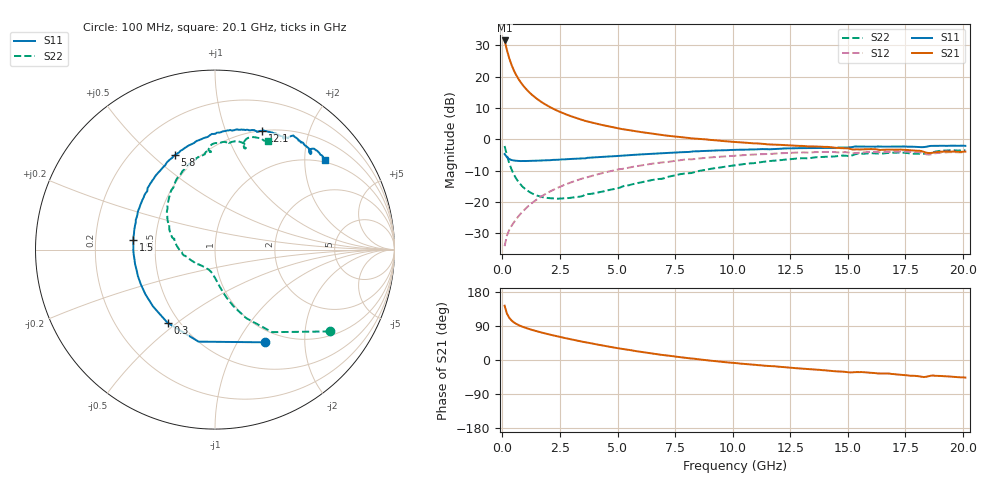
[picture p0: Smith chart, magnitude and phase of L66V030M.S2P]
!  Infineon Technologies AG
! BFR380L3 , PF131585-7, No.6, Th 09.10.01, soldered on pcb-board, measured with PP GSG850
!  Vce=6.0 V,  Ic=30.0 mA
! Common Emitter S-Parameters:  15. November 2001
#  GHz  S  MA  R  50
! f  S11  S21  S12  S22
! GHz  Mag  Ang  Mag  Ang  Mag  Ang  Mag  Ang
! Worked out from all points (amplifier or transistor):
!   201 points, 100 MHz to 20.1 GHz, reference 50 ohm
!   highest |S21| = 31.6 dB at 100 MHz (marker M1)
!   |S21| within 3 dB of that: start of sweep to 198.6 MHz
!   unconditionally stable (mu >= 1): 1.287 GHz to 4.334 GHz
!   at 3.4 GHz: K = 1.02, MAG = 8.7 dB, |S12| = -12.7 dB
!   at 10.1 GHz: K = 0.95, MSG = 2.2 dB, |S12| = -5.2 dB
!   at 20.1 GHz: K = 0.98, MSG = 0.1 dB, |S12| = -4.1 dB
!   S11 on the Smith chart (normalised r, x): 100 MHz: 0.83, -1.31; 300 MHz: 0.43, -0.46; 1.5 GHz: 0.37, +0.05; 5.8 GHz: 0.38, +0.59; 12.1 GHz: 0.50, +1.35; 20.1 GHz: 0.94, +2.51
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0.1  0.5856 -61.9  38.01 143.4  0.01977 63.3  0.7855 -35.5
0.2  0.5209 -100.1  26.78 122.6  0.02924 56.4  0.5593 -55.3
0.3  0.486 -123.0  19.81 111.5  0.03579 56.0  0.4181 -65.6
0.4  0.4685 -137.5  15.52 104.4  0.04163 57.1  0.3319 -71.9
0.5  0.4607 -147.4  12.68 99.3  0.04727 58.9  0.2762 -76.4
0.6  0.4562 -155.1  10.7 95.6  0.05313 60.4  0.2382 -79.6
0.7  0.4542 -161.0  9.258 92.4  0.05923 61.7  0.2101 -82.5
0.8  0.4515 -165.5  8.147 89.6  0.06541 63.0  0.1894 -84.9
1  0.4519 -173.3  6.582 85.0  0.07798 64.4  0.1611 -89.2
1.2  0.455 -179.4  5.519 81.1  0.09076 65.2  0.1435 -93.3
1.5  0.458 173.2  4.455 75.8  0.1103 65.5  0.1273 -99.3
1.8  0.4624 167.0  3.743 71.0  0.1299 65.0  0.1185 -105.5
2.3  0.4718 157.8  2.975 63.7  0.1624 63.3  0.1132 -116.5
2.8  0.4836 149.7  2.484 56.9  0.1946 60.9  0.1154 -126.9
3.5  0.498 139.6  2.029 48.0  0.2394 56.9  0.1254 -139.1
5.8  0.572 113.0  1.352 23.5  0.3723 42.4  0.1983 -179.9
6.8  0.5996 103.5  1.195 14.5  0.4242 35.3  0.2338 166.1
10.1  0.6806 79.0  0.9095 -8.0  0.5508 13.8  0.3869 131.4
12.1  0.7111 68.3  0.8175 -18.1  0.6023 1.6  0.4679 113.4
13.5  0.7289 61.2  0.7732 -24.6  0.6233 -7.1  0.5121 102.6
16.8  0.7683 48.8  0.6881 -35.8  0.6329 -23.5  0.6097 80.5
20.1  0.7903 39.1  0.639 -46.4  0.6265 -37.4  0.6722 63.8
